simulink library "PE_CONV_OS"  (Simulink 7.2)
settings: Solver=ode45  SolverMode=SingleTasking  StartTime=0.0  StopTime=10.0  RelTol=1e-3
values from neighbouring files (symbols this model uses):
  C = 10e-3*1    (= 0.01)    [INIT_B6_2L_3Ph_IGBT_OS.m]    (also in INIT_B6_3L_3Ph_IGBT_OS.m; INIT_MMC_100L.m = 0.005; INIT_MMC_200L.m = 0.005; INIT_MMC_20L.m)
  FS = 900    [INIT_B6_2L_3Ph_IGBT_OS.m]    (also in INIT_B6_3L_3Ph_IGBT_OS.m; INIT_PWM_2L.m = 1000; INIT_PWM_3L.m = 1000; INIT_PWM_Con.m = 1000)
  LN = 2e-3    (= 0.002)    [INIT_PWM_2L.m]    (also in INIT_PWM_3L.m; INIT_PWM_Con.m; INIT_MMC_100L.m = 0.025; INIT_MMC_200L.m = 0.025)
  LS = 1e-3    (= 0.001)    [INIT_B6_2L_3Ph_IGBT_OS.m]    (also in INIT_B6_3L_3Ph_IGBT_OS.m; INIT_MMC_100L.m = 0.025; INIT_MMC_200L.m = 0.025; INIT_MMC_20L.m = 0.0025)
  LT = LN    (= 0.025)    [INIT_MMC_100L.m]    (also in INIT_MMC_200L.m; INIT_MMC_20L.m = 0.002; INIT_MMC_400L.m)
  Nc = 100    [INIT_MMC_100L.m]    (also in INIT_MMC_200L.m = 200; INIT_MMC_20L.m = 20; INIT_MMC_400L.m = 400)
  NT = sqrt(3)*340/400    [INIT_MMC_100L.m]    (also in INIT_MMC_200L.m; INIT_MMC_20L.m = sqrt(3); INIT_MMC_400L.m)
  Rg = 1e-3    (= 0.001)    [INIT_MMC_100L.m]    (also in INIT_MMC_200L.m; INIT_MMC_20L.m; INIT_MMC_400L.m)
  RN = 0.1    [INIT_PWM_2L.m]    (also in INIT_PWM_3L.m; INIT_PWM_Con.m; INIT_MMC_100L.m; INIT_MMC_200L.m)
  RT = RN    (= 0.1)    [INIT_MMC_100L.m]    (also in INIT_MMC_200L.m; INIT_MMC_20L.m; INIT_MMC_400L.m)
  UC0 = 600    [INIT_B6_2L_3Ph_IGBT_OS.m]    (also in INIT_B6_3L_3Ph_IGBT_OS.m = 500; INIT_MMC_100L.m = 6800; INIT_MMC_200L.m = 3400; INIT_MMC_20L.m = 5000)
undefined symbols (not defined in the file or in its folder): A, DT, FT, L, O1, O2, PHT, T, Td
libraries: simulink_extras x2
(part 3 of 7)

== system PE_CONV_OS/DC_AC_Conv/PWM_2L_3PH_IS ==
  Sw : Inport  OutDataType=sfix(16)  OutScaling=2^0
  vDC : Inport  Port=2  OutDataType=sfix(16)  OutScaling=2^0
  I_AB : Inport  Port=3  OutDataType=sfix(16)  OutScaling=2^0
  Mux : Mux  Inputs="[6  1  2]"
  pwm2l_IS_OS : S-Function  FunctionName=s_pwm_2L_3PH_IS_OS  Parameters=0  EnableBusSupport=off
  vABC : Outport  OutDataType=sfix(16)  OutScaling=2^0
  iABC : Outport  Port=2  OutDataType=sfix(16)  OutScaling=2^0
  vAB : Outport  Port=3  OutDataType=sfix(16)  OutScaling=2^0
  iT1,iD1,vT1 : Outport  Port=4  OutDataType=sfix(16)  OutScaling=2^0
  iDC : Outport  Port=5  OutDataType=sfix(16)  OutScaling=2^0
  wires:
  pwm2l_IS_OS/5 -> iDC/1
  pwm2l_IS_OS/3 -> vAB/1
  pwm2l_IS_OS/2 -> iABC/1
  pwm2l_IS_OS/1 -> vABC/1
  pwm2l_IS_OS/4 -> iT1,iD1,vT1/1
  I_AB/1 -> Mux/3
  Mux/1 -> pwm2l_IS_OS/1
  vDC/1 -> Mux/2
  Sw/1 -> Mux/1

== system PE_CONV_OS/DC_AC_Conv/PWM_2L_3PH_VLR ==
  Sw : Inport  OutDataType=sfix(16)  OutScaling=2^0
  vDC : Inport  Port=2  OutDataType=sfix(16)  OutScaling=2^0
  E_ABC : Inport  Port=3  OutDataType=sfix(16)  OutScaling=2^0
  Mux : Mux  Inputs="[6  1  3]"
  pwm2l_VLR_OS : S-Function  FunctionName=s_pwm_2L_3PH_VLR_OS  Parameters="[RL  LL]"  EnableBusSupport=off
  vABC : Outport  OutDataType=sfix(16)  OutScaling=2^0
  iABC : Outport  Port=2  OutDataType=sfix(16)  OutScaling=2^0
  vAB : Outport  Port=3  OutDataType=sfix(16)  OutScaling=2^0
  iT1,iD1,vT1 : Outport  Port=4  OutDataType=sfix(16)  OutScaling=2^0
  iDC : Outport  Port=5  OutDataType=sfix(16)  OutScaling=2^0
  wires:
  Sw/1 -> Mux/1
  vDC/1 -> Mux/2
  Mux/1 -> pwm2l_VLR_OS/1
  E_ABC/1 -> Mux/3
  pwm2l_VLR_OS/4 -> iT1,iD1,vT1/1
  pwm2l_VLR_OS/1 -> vABC/1
  pwm2l_VLR_OS/2 -> iABC/1
  pwm2l_VLR_OS/3 -> vAB/1
  pwm2l_VLR_OS/5 -> iDC/1

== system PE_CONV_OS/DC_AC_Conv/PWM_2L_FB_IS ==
  Sw : Inport  OutDataType=sfix(16)  OutScaling=2^0
  vDC : Inport  Port=2  OutDataType=sfix(16)  OutScaling=2^0
  IS : Inport  Port=3  OutDataType=sfix(16)  OutScaling=2^0
  Mux : Mux  Inputs="[4  1  1]"
  pwm2l_FB_IS_OS : S-Function  FunctionName=s_pwm_2L_FB_IS_OS  Parameters=0  EnableBusSupport=off
  vA : Outport  OutDataType=sfix(16)  OutScaling=2^0
  iA : Outport  Port=2  OutDataType=sfix(16)  OutScaling=2^0
  vAB : Outport  Port=3  OutDataType=sfix(16)  OutScaling=2^0
  iT1,iD1,vT1 : Outport  Port=4  OutDataType=sfix(16)  OutScaling=2^0
  iDC : Outport  Port=5  OutDataType=sfix(16)  OutScaling=2^0
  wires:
  pwm2l_FB_IS_OS/5 -> iDC/1
  Sw/1 -> Mux/1
  vDC/1 -> Mux/2
  Mux/1 -> pwm2l_FB_IS_OS/1
  IS/1 -> Mux/3
  pwm2l_FB_IS_OS/1 -> vA/1
  pwm2l_FB_IS_OS/2 -> iA/1
  pwm2l_FB_IS_OS/3 -> vAB/1
  pwm2l_FB_IS_OS/4 -> iT1,iD1,vT1/1

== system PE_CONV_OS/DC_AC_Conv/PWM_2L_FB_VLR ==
  Sw : Inport  OutDataType=sfix(16)  OutScaling=2^0
  vDC : Inport  Port=2  OutDataType=sfix(16)  OutScaling=2^0
  EA : Inport  Port=3  OutDataType=sfix(16)  OutScaling=2^0
  Mux : Mux  Inputs="[4  1  1]"
  pwm2l_FB_IS_OS : S-Function  FunctionName=s_pwm_2L_FB_VLR_OS  Parameters="[RL  LL]"  EnableBusSupport=off
  vA : Outport  OutDataType=sfix(16)  OutScaling=2^0
  iA1 : Outport  Port=2  OutDataType=sfix(16)  OutScaling=2^0
  vAB : Outport  Port=3  OutDataType=sfix(16)  OutScaling=2^0
  iT1,iD1,vT1 : Outport  Port=4  OutDataType=sfix(16)  OutScaling=2^0
  iDC : Outport  Port=5  OutDataType=sfix(16)  OutScaling=2^0
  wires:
  pwm2l_FB_IS_OS/5 -> iDC/1
  Sw/1 -> Mux/1
  vDC/1 -> Mux/2
  Mux/1 -> pwm2l_FB_IS_OS/1
  EA/1 -> Mux/3
  pwm2l_FB_IS_OS/1 -> vA/1
  pwm2l_FB_IS_OS/2 -> iA1/1
  pwm2l_FB_IS_OS/3 -> vAB/1
  pwm2l_FB_IS_OS/4 -> iT1,iD1,vT1/1

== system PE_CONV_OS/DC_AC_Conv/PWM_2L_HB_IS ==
  Sw : Inport  OutDataType=sfix(16)  OutScaling=2^0
  vDC : Inport  Port=2  OutDataType=sfix(16)  OutScaling=2^0
  IS : Inport  Port=3  OutDataType=sfix(16)  OutScaling=2^0
  Mux : Mux  Inputs="[2  1  1]"
  pwm2l_HB_IS_OS : S-Function  FunctionName=s_pwm_2L_HB_IS_OS  Parameters=0  EnableBusSupport=off
  vA : Outport  OutDataType=sfix(16)  OutScaling=2^0
  iA : Outport  Port=2  OutDataType=sfix(16)  OutScaling=2^0
  iT1,iD1,vT1 : Outport  Port=3  OutDataType=sfix(16)  OutScaling=2^0
  iDC : Outport  Port=4  OutDataType=sfix(16)  OutScaling=2^0
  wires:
  Sw/1 -> Mux/1
  vDC/1 -> Mux/2
  Mux/1 -> pwm2l_HB_IS_OS/1
  IS/1 -> Mux/3
  pwm2l_HB_IS_OS/1 -> vA/1
  pwm2l_HB_IS_OS/2 -> iA/1
  pwm2l_HB_IS_OS/3 -> iT1,iD1,vT1/1
  pwm2l_HB_IS_OS/4 -> iDC/1

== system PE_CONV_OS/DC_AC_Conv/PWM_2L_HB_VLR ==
  Sw : Inport  OutDataType=sfix(16)  OutScaling=2^0
  vDC : Inport  Port=2  OutDataType=sfix(16)  OutScaling=2^0
  EA : Inport  Port=3  OutDataType=sfix(16)  OutScaling=2^0
  Mux : Mux  Inputs="[2  1  1]"
  pwm2l_HB_VLR_OS : S-Function  FunctionName=s_pwm_2L_HB_VLR_OS  Parameters="[RL  LL]"  EnableBusSupport=off
  vA : Outport  OutDataType=sfix(16)  OutScaling=2^0
  iA : Outport  Port=2  OutDataType=sfix(16)  OutScaling=2^0
  iT1,iD1,vT1 : Outport  Port=3  OutDataType=sfix(16)  OutScaling=2^0
  iDC : Outport  Port=4  OutDataType=sfix(16)  OutScaling=2^0
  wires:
  Sw/1 -> Mux/1
  vDC/1 -> Mux/2
  Mux/1 -> pwm2l_HB_VLR_OS/1
  EA/1 -> Mux/3
  pwm2l_HB_VLR_OS/1 -> vA/1
  pwm2l_HB_VLR_OS/2 -> iA/1
  pwm2l_HB_VLR_OS/3 -> iT1,iD1,vT1/1
  pwm2l_HB_VLR_OS/4 -> iDC/1

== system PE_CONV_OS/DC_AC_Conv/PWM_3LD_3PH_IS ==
  Sw : Inport  OutDataType=sfix(16)  OutScaling=2^0
  vDC : Inport  Port=2  OutDataType=sfix(16)  OutScaling=2^0
  I_AB : Inport  Port=3  OutDataType=sfix(16)  OutScaling=2^0
  Mux : Mux  Inputs="[12  1  2]"
  pwm3LD_OS : S-Function  FunctionName=s_pwm_3LD_3PH_IS_OS  Parameters=0  EnableBusSupport=off
  vABC : Outport  OutDataType=sfix(16)  OutScaling=2^0
  iABC : Outport  Port=2  OutDataType=sfix(16)  OutScaling=2^0
  vAB : Outport  Port=3  OutDataType=sfix(16)  OutScaling=2^0
  "iT1, iD1,vT1" : Outport  Port=4  OutDataType=sfix(16)  OutScaling=2^0
  "iT2, iD2,vT2" : Outport  Port=5  OutDataType=sfix(16)  OutScaling=2^0
  iD5,vD5 : Outport  Port=6  OutDataType=sfix(16)  OutScaling=2^0
  iDC1,iDC2 : Outport  Port=7  OutDataType=sfix(16)  OutScaling=2^0
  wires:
  pwm3LD_OS/7 -> iDC1,iDC2/1
  pwm3LD_OS/6 -> iD5,vD5/1
  pwm3LD_OS/5 -> "iT2, iD2,vT2"/1
  pwm3LD_OS/3 -> vAB/1
  pwm3LD_OS/2 -> iABC/1
  pwm3LD_OS/4 -> "iT1, iD1,vT1"/1
  pwm3LD_OS/1 -> vABC/1
  I_AB/1 -> Mux/3
  Mux/1 -> pwm3LD_OS/1
  vDC/1 -> Mux/2
  Sw/1 -> Mux/1

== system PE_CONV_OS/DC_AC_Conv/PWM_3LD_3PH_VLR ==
  Sw : Inport  OutDataType=sfix(16)  OutScaling=2^0
  vDC : Inport  Port=2  OutDataType=sfix(16)  OutScaling=2^0
  E_ABC : Inport  Port=3  OutDataType=sfix(16)  OutScaling=2^0
  Mux : Mux  Inputs="[12 1  3]"
  pwm3LD_3PH_VLR_OS : S-Function  FunctionName=s_pwm_3LD_3PH_VLR_OS  Parameters="[RL  LL]"  EnableBusSupport=off
  vABC : Outport  OutDataType=sfix(16)  OutScaling=2^0
  iABC : Outport  Port=2  OutDataType=sfix(16)  OutScaling=2^0
  vAB : Outport  Port=3  OutDataType=sfix(16)  OutScaling=2^0
  "iT1, iD1,vT1" : Outport  Port=4  OutDataType=sfix(16)  OutScaling=2^0
  "iT2, iD2,vT2" : Outport  Port=5  OutDataType=sfix(16)  OutScaling=2^0
  iD5,vD5 : Outport  Port=6  OutDataType=sfix(16)  OutScaling=2^0
  iDC1,iDC2 : Outport  Port=7  OutDataType=sfix(16)  OutScaling=2^0
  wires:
  Sw/1 -> Mux/1
  vDC/1 -> Mux/2
  Mux/1 -> pwm3LD_3PH_VLR_OS/1
  E_ABC/1 -> Mux/3
  pwm3LD_3PH_VLR_OS/1 -> vABC/1
  pwm3LD_3PH_VLR_OS/4 -> "iT1, iD1,vT1"/1
  pwm3LD_3PH_VLR_OS/2 -> iABC/1
  pwm3LD_3PH_VLR_OS/3 -> vAB/1
  pwm3LD_3PH_VLR_OS/5 -> "iT2, iD2,vT2"/1
  pwm3LD_3PH_VLR_OS/6 -> iD5,vD5/1
  pwm3LD_3PH_VLR_OS/7 -> iDC1,iDC2/1

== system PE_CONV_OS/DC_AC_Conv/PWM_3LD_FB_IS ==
  Sw : Inport  OutDataType=sfix(16)  OutScaling=2^0
  vDC : Inport  Port=2  OutDataType=sfix(16)  OutScaling=2^0
  iS : Inport  Port=3  OutDataType=sfix(16)  OutScaling=2^0
  Mux : Mux  Inputs="[8  1  1]"
  pwm3LD_IS_OS : S-Function  FunctionName=s_pwm_3LD_FB_IS_OS  Parameters=0  EnableBusSupport=off
  vA : Outport  OutDataType=sfix(16)  OutScaling=2^0
  iA : Outport  Port=2  OutDataType=sfix(16)  OutScaling=2^0
  vAB : Outport  Port=3  OutDataType=sfix(16)  OutScaling=2^0
  "iT1, iD1,vT1" : Outport  Port=4  OutDataType=sfix(16)  OutScaling=2^0
  "iT2, iD2,vT2" : Outport  Port=5  OutDataType=sfix(16)  OutScaling=2^0
  iD5,vD5 : Outport  Port=6  OutDataType=sfix(16)  OutScaling=2^0
  iDC1,iDC2 : Outport  Port=7  OutDataType=sfix(16)  OutScaling=2^0
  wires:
  pwm3LD_IS_OS/2 -> iA/1
  pwm3LD_IS_OS/3 -> vAB/1
  pwm3LD_IS_OS/4 -> "iT1, iD1,vT1"/1
  pwm3LD_IS_OS/5 -> "iT2, iD2,vT2"/1
  pwm3LD_IS_OS/6 -> iD5,vD5/1
  pwm3LD_IS_OS/7 -> iDC1,iDC2/1
  Sw/1 -> Mux/1
  vDC/1 -> Mux/2
  Mux/1 -> pwm3LD_IS_OS/1
  iS/1 -> Mux/3
  pwm3LD_IS_OS/1 -> vA/1

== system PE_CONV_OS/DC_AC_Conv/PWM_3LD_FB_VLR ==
  Sw : Inport  OutDataType=sfix(16)  OutScaling=2^0
  vDC : Inport  Port=2  OutDataType=sfix(16)  OutScaling=2^0
  E_A : Inport  Port=3  OutDataType=sfix(16)  OutScaling=2^0
  Mux : Mux  Inputs="[8  1  1]"
  pwm3LD_VLR_OS : S-Function  FunctionName=s_pwm_3LD_FB_VLR_OS  Parameters="[RL  LL]"  EnableBusSupport=off
  vA : Outport  OutDataType=sfix(16)  OutScaling=2^0
  iA : Outport  Port=2  OutDataType=sfix(16)  OutScaling=2^0
  vAB : Outport  Port=3  OutDataType=sfix(16)  OutScaling=2^0
  "iT1, iD1,vT1" : Outport  Port=4  OutDataType=sfix(16)  OutScaling=2^0
  "iT2, iD2,vT2" : Outport  Port=5  OutDataType=sfix(16)  OutScaling=2^0
  iD5,vD5 : Outport  Port=6  OutDataType=sfix(16)  OutScaling=2^0
  iDC1,iDC2 : Outport  Port=7  OutDataType=sfix(16)  OutScaling=2^0
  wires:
  pwm3LD_VLR_OS/7 -> iDC1,iDC2/1
  pwm3LD_VLR_OS/6 -> iD5,vD5/1
  pwm3LD_VLR_OS/5 -> "iT2, iD2,vT2"/1
  pwm3LD_VLR_OS/4 -> "iT1, iD1,vT1"/1
  pwm3LD_VLR_OS/3 -> vAB/1
  pwm3LD_VLR_OS/2 -> iA/1
  pwm3LD_VLR_OS/1 -> vA/1
  E_A/1 -> Mux/3
  Mux/1 -> pwm3LD_VLR_OS/1
  vDC/1 -> Mux/2
  Sw/1 -> Mux/1

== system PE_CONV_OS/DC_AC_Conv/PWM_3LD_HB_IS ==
  Sw : Inport  OutDataType=sfix(16)  OutScaling=2^0
  vDC : Inport  Port=2  OutDataType=sfix(16)  OutScaling=2^0
  iS : Inport  Port=3  OutDataType=sfix(16)  OutScaling=2^0
  Mux : Mux  Inputs="[4  1  1]"
  pwm3LD_HB_IS_OS : S-Function  FunctionName=s_pwm_3LD_HB_IS_OS  Parameters=0  EnableBusSupport=off
  vA : Outport  OutDataType=sfix(16)  OutScaling=2^0
  iA : Outport  Port=2  OutDataType=sfix(16)  OutScaling=2^0
  "iT1, iD1,vT1" : Outport  Port=3  OutDataType=sfix(16)  OutScaling=2^0
  "iT2, iD2,vT2" : Outport  Port=4  OutDataType=sfix(16)  OutScaling=2^0
  iD5,vD5 : Outport  Port=5  OutDataType=sfix(16)  OutScaling=2^0
  iDC1,iDC2 : Outport  Port=6  OutDataType=sfix(16)  OutScaling=2^0
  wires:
  pwm3LD_HB_IS_OS/6 -> iDC1,iDC2/1
  pwm3LD_HB_IS_OS/1 -> vA/1
  iS/1 -> Mux/3
  Mux/1 -> pwm3LD_HB_IS_OS/1
  vDC/1 -> Mux/2
  Sw/1 -> Mux/1
  pwm3LD_HB_IS_OS/2 -> iA/1
  pwm3LD_HB_IS_OS/3 -> "iT1, iD1,vT1"/1
  pwm3LD_HB_IS_OS/4 -> "iT2, iD2,vT2"/1
  pwm3LD_HB_IS_OS/5 -> iD5,vD5/1

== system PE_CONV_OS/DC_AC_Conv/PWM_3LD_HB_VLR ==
  Sw : Inport  OutDataType=sfix(16)  OutScaling=2^0
  vDC : Inport  Port=2  OutDataType=sfix(16)  OutScaling=2^0
  EA : Inport  Port=3  OutDataType=sfix(16)  OutScaling=2^0
  Mux : Mux  Inputs="[4  1 1]"
  pwm3LD_HB_VLR_OS : S-Function  FunctionName=s_pwm_3LD_HB_VLR_OS  Parameters="[RL  LL]"  EnableBusSupport=off
  vA : Outport  OutDataType=sfix(16)  OutScaling=2^0
  iA : Outport  Port=2  OutDataType=sfix(16)  OutScaling=2^0
  "iT1, iD1,vT1" : Outport  Port=3  OutDataType=sfix(16)  OutScaling=2^0
  "iT2, iD2,vT2" : Outport  Port=4  OutDataType=sfix(16)  OutScaling=2^0
  iD5,vD5 : Outport  Port=5  OutDataType=sfix(16)  OutScaling=2^0
  iDC1,iDC2 : Outport  Port=6  OutDataType=sfix(16)  OutScaling=2^0
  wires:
  Sw/1 -> Mux/1
  vDC/1 -> Mux/2
  Mux/1 -> pwm3LD_HB_VLR_OS/1
  EA/1 -> Mux/3
  pwm3LD_HB_VLR_OS/1 -> vA/1
  pwm3LD_HB_VLR_OS/2 -> iA/1
  pwm3LD_HB_VLR_OS/3 -> "iT1, iD1,vT1"/1
  pwm3LD_HB_VLR_OS/4 -> "iT2, iD2,vT2"/1
  pwm3LD_HB_VLR_OS/5 -> iD5,vD5/1
  pwm3LD_HB_VLR_OS/6 -> iDC1,iDC2/1

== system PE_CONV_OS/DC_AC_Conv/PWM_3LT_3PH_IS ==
  Sw : Inport  OutDataType=sfix(16)  OutScaling=2^0
  vDC : Inport  Port=2  OutDataType=sfix(16)  OutScaling=2^0
  I_AB : Inport  Port=3  OutDataType=sfix(16)  OutScaling=2^0
  Mux : Mux  Inputs="[12  1  2]"
  pwm3LD_OS : S-Function  FunctionName=s_pwm_3LT_3PH_IS_OS  Parameters=0  EnableBusSupport=off
  vABC : Outport  OutDataType=sfix(16)  OutScaling=2^0
  iABC : Outport  Port=2  OutDataType=sfix(16)  OutScaling=2^0
  vAB : Outport  Port=3  OutDataType=sfix(16)  OutScaling=2^0
  "iT1, iD1,vT1" : Outport  Port=4  OutDataType=sfix(16)  OutScaling=2^0
  "iT2, iD2,vT2" : Outport  Port=5  OutDataType=sfix(16)  OutScaling=2^0
  iDC1,iDC2 : Outport  Port=6  OutDataType=sfix(16)  OutScaling=2^0
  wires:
  Sw/1 -> Mux/1
  vDC/1 -> Mux/2
  Mux/1 -> pwm3LD_OS/1
  I_AB/1 -> Mux/3
  pwm3LD_OS/1 -> vABC/1
  pwm3LD_OS/4 -> "iT1, iD1,vT1"/1
  pwm3LD_OS/2 -> iABC/1
  pwm3LD_OS/3 -> vAB/1
  pwm3LD_OS/5 -> "iT2, iD2,vT2"/1
  pwm3LD_OS/6 -> iDC1,iDC2/1

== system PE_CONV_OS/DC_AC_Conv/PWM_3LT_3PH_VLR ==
  Sw : Inport  OutDataType=sfix(16)  OutScaling=2^0
  vDC : Inport  Port=2  OutDataType=sfix(16)  OutScaling=2^0
  E_ABC : Inport  Port=3  OutDataType=sfix(16)  OutScaling=2^0
  Mux : Mux  Inputs="[12 1  3]"
  pwm3LD_3PH_VLR_OS : S-Function  FunctionName=s_pwm_3LT_3PH_VLR_OS  Parameters="[RL  LL]"  EnableBusSupport=off
  vABC : Outport  OutDataType=sfix(16)  OutScaling=2^0
  iABC : Outport  Port=2  OutDataType=sfix(16)  OutScaling=2^0
  vAB : Outport  Port=3  OutDataType=sfix(16)  OutScaling=2^0
  "iT1, iD1,vT1" : Outport  Port=4  OutDataType=sfix(16)  OutScaling=2^0
  "iT2, iD2,vT2" : Outport  Port=5  OutDataType=sfix(16)  OutScaling=2^0
  iDC1,iDC2 : Outport  Port=6  OutDataType=sfix(16)  OutScaling=2^0
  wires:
  pwm3LD_3PH_VLR_OS/6 -> iDC1,iDC2/1
  pwm3LD_3PH_VLR_OS/5 -> "iT2, iD2,vT2"/1
  pwm3LD_3PH_VLR_OS/3 -> vAB/1
  pwm3LD_3PH_VLR_OS/2 -> iABC/1
  pwm3LD_3PH_VLR_OS/4 -> "iT1, iD1,vT1"/1
  pwm3LD_3PH_VLR_OS/1 -> vABC/1
  E_ABC/1 -> Mux/3
  Mux/1 -> pwm3LD_3PH_VLR_OS/1
  vDC/1 -> Mux/2
  Sw/1 -> Mux/1

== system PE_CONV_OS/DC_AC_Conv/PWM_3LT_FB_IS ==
  Sw : Inport  OutDataType=sfix(16)  OutScaling=2^0
  vDC : Inport  Port=2  OutDataType=sfix(16)  OutScaling=2^0
  IS : Inport  Port=3  OutDataType=sfix(16)  OutScaling=2^0
  Mux : Mux  Inputs="[8 1  1]"
  pwm3LD_IS_OS : S-Function  FunctionName=s_pwm_3LT_FB_IS_OS  Parameters=[0]  EnableBusSupport=off
  vA : Outport  OutDataType=sfix(16)  OutScaling=2^0
  IA : Outport  Port=2  OutDataType=sfix(16)  OutScaling=2^0
  vAB : Outport  Port=3  OutDataType=sfix(16)  OutScaling=2^0
  "iT1, iD1,vT1" : Outport  Port=4  OutDataType=sfix(16)  OutScaling=2^0
  "iT2, iD2,vT2" : Outport  Port=5  OutDataType=sfix(16)  OutScaling=2^0
  iDC1,iDC2 : Outport  Port=6  OutDataType=sfix(16)  OutScaling=2^0
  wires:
  pwm3LD_IS_OS/6 -> iDC1,iDC2/1
  pwm3LD_IS_OS/5 -> "iT2, iD2,vT2"/1
  pwm3LD_IS_OS/4 -> "iT1, iD1,vT1"/1
  pwm3LD_IS_OS/3 -> vAB/1
  pwm3LD_IS_OS/2 -> IA/1
  Sw/1 -> Mux/1
  vDC/1 -> Mux/2
  Mux/1 -> pwm3LD_IS_OS/1
  IS/1 -> Mux/3
  pwm3LD_IS_OS/1 -> vA/1

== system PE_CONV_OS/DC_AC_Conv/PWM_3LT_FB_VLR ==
  Sw : Inport  OutDataType=sfix(16)  OutScaling=2^0
  vDC : Inport  Port=2  OutDataType=sfix(16)  OutScaling=2^0
  E_A : Inport  Port=3  OutDataType=sfix(16)  OutScaling=2^0
  Mux : Mux  Inputs="[8  1  1]"
  pwm3LD_VLR_OS : S-Function  FunctionName=s_pwm_3LT_FB_VLR_OS  Parameters="[RL  LL]"  EnableBusSupport=off
  vA : Outport  OutDataType=sfix(16)  OutScaling=2^0
  iA : Outport  Port=2  OutDataType=sfix(16)  OutScaling=2^0
  vAB : Outport  Port=3  OutDataType=sfix(16)  OutScaling=2^0
  "iT1, iD1,vT1" : Outport  Port=4  OutDataType=sfix(16)  OutScaling=2^0
  "iT2, iD2,vT2" : Outport  Port=5  OutDataType=sfix(16)  OutScaling=2^0
  "iDC1, iDC2" : Outport  Port=6  OutDataType=sfix(16)  OutScaling=2^0
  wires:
  pwm3LD_VLR_OS/6 -> "iDC1, iDC2"/1
  Sw/1 -> Mux/1
  vDC/1 -> Mux/2
  Mux/1 -> pwm3LD_VLR_OS/1
  E_A/1 -> Mux/3
  pwm3LD_VLR_OS/1 -> vA/1
  pwm3LD_VLR_OS/2 -> iA/1
  pwm3LD_VLR_OS/3 -> vAB/1
  pwm3LD_VLR_OS/4 -> "iT1, iD1,vT1"/1
  pwm3LD_VLR_OS/5 -> "iT2, iD2,vT2"/1

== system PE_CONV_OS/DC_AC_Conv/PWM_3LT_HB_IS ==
  Sw : Inport  OutDataType=sfix(16)  OutScaling=2^0
  vDC : Inport  Port=2  OutDataType=sfix(16)  OutScaling=2^0
  iS : Inport  Port=3  OutDataType=sfix(16)  OutScaling=2^0
  Mux : Mux  Inputs="[4  1  1]"
  pwm3LT_HB_IS_OS : S-Function  FunctionName=s_pwm_3LT_HB_IS_OS  Parameters=0  EnableBusSupport=off
  vA : Outport  OutDataType=sfix(16)  OutScaling=2^0
  iA : Outport  Port=2  OutDataType=sfix(16)  OutScaling=2^0
  "iT1, iD1,vT1" : Outport  Port=3  OutDataType=sfix(16)  OutScaling=2^0
  "iT2, iD2,vT2" : Outport  Port=4  OutDataType=sfix(16)  OutScaling=2^0
  iDC1,iDC2 : Outport  Port=5  OutDataType=sfix(16)  OutScaling=2^0
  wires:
  pwm3LT_HB_IS_OS/5 -> iDC1,iDC2/1
  pwm3LT_HB_IS_OS/4 -> "iT2, iD2,vT2"/1
  pwm3LT_HB_IS_OS/3 -> "iT1, iD1,vT1"/1
  pwm3LT_HB_IS_OS/2 -> iA/1
  Sw/1 -> Mux/1
  vDC/1 -> Mux/2
  Mux/1 -> pwm3LT_HB_IS_OS/1
  iS/1 -> Mux/3
  pwm3LT_HB_IS_OS/1 -> vA/1

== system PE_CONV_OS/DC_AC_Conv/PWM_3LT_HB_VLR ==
  Sw : Inport  OutDataType=sfix(16)  OutScaling=2^0
  vDC : Inport  Port=2  OutDataType=sfix(16)  OutScaling=2^0
  EA : Inport  Port=3  OutDataType=sfix(16)  OutScaling=2^0
  Mux : Mux  Inputs="[4  1 1]"
  pwm3LD_HB_VLR_OS : S-Function  FunctionName=s_pwm_3LT_HB_VLR_OS  Parameters="[RL  LL]"  EnableBusSupport=off
  vA : Outport  OutDataType=sfix(16)  OutScaling=2^0
  iA : Outport  Port=2  OutDataType=sfix(16)  OutScaling=2^0
  "iT1, iD1,vT1" : Outport  Port=3  OutDataType=sfix(16)  OutScaling=2^0
  "iT2, iD2,vT2" : Outport  Port=4  OutDataType=sfix(16)  OutScaling=2^0
  iDC1,iDC2 : Outport  Port=5  OutDataType=sfix(16)  OutScaling=2^0
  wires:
  pwm3LD_HB_VLR_OS/5 -> iDC1,iDC2/1
  pwm3LD_HB_VLR_OS/4 -> "iT2, iD2,vT2"/1
  pwm3LD_HB_VLR_OS/3 -> "iT1, iD1,vT1"/1
  pwm3LD_HB_VLR_OS/2 -> iA/1
  pwm3LD_HB_VLR_OS/1 -> vA/1
  EA/1 -> Mux/3
  Mux/1 -> pwm3LD_HB_VLR_OS/1
  vDC/1 -> Mux/2
  Sw/1 -> Mux/1

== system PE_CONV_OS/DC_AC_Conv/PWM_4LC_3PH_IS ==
  Sw : Inport  OutDataType=sfix(16)  OutScaling=2^0
  vDC : Inport  Port=2  OutDataType=sfix(16)  OutScaling=2^0
  i_AB : Inport  Port=3  OutDataType=sfix(16)  OutScaling=2^0
  Mux : Mux  Inputs="[18  1  2]"
  pwm3LD_3PH_IS_OS : S-Function  FunctionName=s_pwm_4LC_3PH_IS_OS  Parameters="[C1  VC10  C2  VC20]"  EnableBusSupport=off
  vABC : Outport  OutDataType=sfix(16)  OutScaling=2^0
  iABC : Outport  Port=2  OutDataType=sfix(16)  OutScaling=2^0
  vAB : Outport  Port=3  OutDataType=sfix(16)  OutScaling=2^0
  iT1,iD1,vT1 : Outport  Port=4  OutDataType=sfix(16)  OutScaling=2^0
  iT2,ID2,vT2 : Outport  Port=5  OutDataType=sfix(16)  OutScaling=2^0
  iT3,iD3,vT3 : Outport  Port=6  OutDataType=sfix(16)  OutScaling=2^0
  iDC1,IDC2 : Outport  Port=7  OutDataType=sfix(16)  OutScaling=2^0
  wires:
  pwm3LD_3PH_IS_OS/6 -> iT3,iD3,vT3/1
  pwm3LD_3PH_IS_OS/5 -> iT2,ID2,vT2/1
  pwm3LD_3PH_IS_OS/4 -> iT1,iD1,vT1/1
  pwm3LD_3PH_IS_OS/3 -> vAB/1
  Sw/1 -> Mux/1
  vDC/1 -> Mux/2
  Mux/1 -> pwm3LD_3PH_IS_OS/1
  i_AB/1 -> Mux/3
  pwm3LD_3PH_IS_OS/1 -> vABC/1
  pwm3LD_3PH_IS_OS/2 -> iABC/1
  pwm3LD_3PH_IS_OS/7 -> iDC1,IDC2/1

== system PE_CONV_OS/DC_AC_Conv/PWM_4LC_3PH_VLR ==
  Sw : Inport  OutDataType=sfix(16)  OutScaling=2^0
  vDC : Inport  Port=2  OutDataType=sfix(16)  OutScaling=2^0
  E_ABC : Inport  Port=3  OutDataType=sfix(16)  OutScaling=2^0
  Mux : Mux  Inputs="[18  1  3]"
  pwm3LD_3PH_VLR_OS : S-Function  FunctionName=s_pwm_4LC_3PH_VLR_OS  Parameters="[C1  VC10  C2  VC20  RL  LL]"  EnableBusSupport=off
  vABC : Outport  OutDataType=sfix(16)  OutScaling=2^0
  iABC : Outport  Port=2  OutDataType=sfix(16)  OutScaling=2^0
  vAB : Outport  Port=3  OutDataType=sfix(16)  OutScaling=2^0
  iT1,iD1,vT1 : Outport  Port=4  OutDataType=sfix(16)  OutScaling=2^0
  iT2,ID2,vT2 : Outport  Port=5  OutDataType=sfix(16)  OutScaling=2^0
  iT3,iD3,vT3 : Outport  Port=6  OutDataType=sfix(16)  OutScaling=2^0
  iDC1. iDC2 : Outport  Port=7  OutDataType=sfix(16)  OutScaling=2^0
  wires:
  pwm3LD_3PH_VLR_OS/7 -> iDC1. iDC2/1
  pwm3LD_3PH_VLR_OS/2 -> iABC/1
  pwm3LD_3PH_VLR_OS/1 -> vABC/1
  E_ABC/1 -> Mux/3
  Mux/1 -> pwm3LD_3PH_VLR_OS/1
  vDC/1 -> Mux/2
  Sw/1 -> Mux/1
  pwm3LD_3PH_VLR_OS/3 -> vAB/1
  pwm3LD_3PH_VLR_OS/4 -> iT1,iD1,vT1/1
  pwm3LD_3PH_VLR_OS/5 -> iT2,ID2,vT2/1
  pwm3LD_3PH_VLR_OS/6 -> iT3,iD3,vT3/1

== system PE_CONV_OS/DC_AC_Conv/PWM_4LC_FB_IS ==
  Sw : Inport  OutDataType=sfix(16)  OutScaling=2^0
  vDC : Inport  Port=2  OutDataType=sfix(16)  OutScaling=2^0
  i_A : Inport  Port=3  OutDataType=sfix(16)  OutScaling=2^0
  Mux : Mux  Inputs="[12  1  1]"
  pwm4Lc_HB_IS_OS : S-Function  FunctionName=s_pwm_4LC_FB_IS_OS  Parameters="[C1  VC10  C2  VC20]"  EnableBusSupport=off
  vA : Outport  OutDataType=sfix(16)  OutScaling=2^0
  iA : Outport  Port=2  OutDataType=sfix(16)  OutScaling=2^0
  iT1,iD1,vT1 : Outport  Port=3  OutDataType=sfix(16)  OutScaling=2^0
  iT2,ID2,vT2 : Outport  Port=4  OutDataType=sfix(16)  OutScaling=2^0
  iT3,iD3,vT3 : Outport  Port=5  OutDataType=sfix(16)  OutScaling=2^0
  iDC1,IDC2 : Outport  Port=6  OutDataType=sfix(16)  OutScaling=2^0
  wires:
  pwm4Lc_HB_IS_OS/5 -> iT3,iD3,vT3/1
  pwm4Lc_HB_IS_OS/4 -> iT2,ID2,vT2/1
  pwm4Lc_HB_IS_OS/3 -> iT1,iD1,vT1/1
  Sw/1 -> Mux/1
  vDC/1 -> Mux/2
  Mux/1 -> pwm4Lc_HB_IS_OS/1
  i_A/1 -> Mux/3
  pwm4Lc_HB_IS_OS/1 -> vA/1
  pwm4Lc_HB_IS_OS/2 -> iA/1
  pwm4Lc_HB_IS_OS/6 -> iDC1,IDC2/1

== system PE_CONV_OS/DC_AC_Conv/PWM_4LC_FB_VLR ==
  Sw : Inport  OutDataType=sfix(16)  OutScaling=2^0
  vDC : Inport  Port=2  OutDataType=sfix(16)  OutScaling=2^0
  VL : Inport  Port=3  OutDataType=sfix(16)  OutScaling=2^0
  Mux : Mux  Inputs="[12  1  1]"
  pwm4Lc_HB_IS_OS : S-Function  FunctionName=s_pwm_4LC_FB_VLR_OS  Parameters="[C1  VC10  C2  VC20 R1 L1]"  EnableBusSupport=off
  vA : Outport  OutDataType=sfix(16)  OutScaling=2^0
  iA : Outport  Port=2  OutDataType=sfix(16)  OutScaling=2^0
  iT1,iD1,vT1 : Outport  Port=3  OutDataType=sfix(16)  OutScaling=2^0
  iT2,ID2,vT2 : Outport  Port=4  OutDataType=sfix(16)  OutScaling=2^0
  iT3,iD3,vT3 : Outport  Port=5  OutDataType=sfix(16)  OutScaling=2^0
  iDC1,IDC2 : Outport  Port=6  OutDataType=sfix(16)  OutScaling=2^0
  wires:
  pwm4Lc_HB_IS_OS/5 -> iT3,iD3,vT3/1
  pwm4Lc_HB_IS_OS/4 -> iT2,ID2,vT2/1
  pwm4Lc_HB_IS_OS/3 -> iT1,iD1,vT1/1
  Sw/1 -> Mux/1
  vDC/1 -> Mux/2
  Mux/1 -> pwm4Lc_HB_IS_OS/1
  VL/1 -> Mux/3
  pwm4Lc_HB_IS_OS/1 -> vA/1
  pwm4Lc_HB_IS_OS/2 -> iA/1
  pwm4Lc_HB_IS_OS/6 -> iDC1,IDC2/1

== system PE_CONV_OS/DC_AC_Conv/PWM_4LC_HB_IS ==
  Sw : Inport  OutDataType=sfix(16)  OutScaling=2^0
  vDC : Inport  Port=2  OutDataType=sfix(16)  OutScaling=2^0
  i_A : Inport  Port=3  OutDataType=sfix(16)  OutScaling=2^0
  Mux : Mux  Inputs="[6  1  1]"
  pwm4Lc_HB_IS_OS : S-Function  FunctionName=s_pwm_4LC_HB_IS_OS  Parameters="[C1  VC10  C2  VC20]"  EnableBusSupport=off
  vA : Outport  OutDataType=sfix(16)  OutScaling=2^0
  iA : Outport  Port=2  OutDataType=sfix(16)  OutScaling=2^0
  iT1,iD1,vT1 : Outport  Port=3  OutDataType=sfix(16)  OutScaling=2^0
  iT2,ID2,vT2 : Outport  Port=4  OutDataType=sfix(16)  OutScaling=2^0
  iT3,iD3,vT3 : Outport  Port=5  OutDataType=sfix(16)  OutScaling=2^0
  iDC1,IDC2 : Outport  Port=6  OutDataType=sfix(16)  OutScaling=2^0
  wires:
  pwm4Lc_HB_IS_OS/5 -> iT3,iD3,vT3/1
  pwm4Lc_HB_IS_OS/4 -> iT2,ID2,vT2/1
  pwm4Lc_HB_IS_OS/3 -> iT1,iD1,vT1/1
  Sw/1 -> Mux/1
  vDC/1 -> Mux/2
  Mux/1 -> pwm4Lc_HB_IS_OS/1
  i_A/1 -> Mux/3
  pwm4Lc_HB_IS_OS/1 -> vA/1
  pwm4Lc_HB_IS_OS/2 -> iA/1
  pwm4Lc_HB_IS_OS/6 -> iDC1,IDC2/1

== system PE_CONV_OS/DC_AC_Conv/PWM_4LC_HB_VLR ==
  Sw : Inport  OutDataType=sfix(16)  OutScaling=2^0
  vDC : Inport  Port=2  OutDataType=sfix(16)  OutScaling=2^0
  vL : Inport  Port=3  OutDataType=sfix(16)  OutScaling=2^0
  Mux : Mux  Inputs="[6  1  1]"
  pwm4Lc_HB_IS_OS : S-Function  FunctionName=s_pwm_4LC_HB_VLR_OS  Parameters="[C1  VC10  C2  VC20 R1  L1]"  EnableBusSupport=off
  vA : Outport  OutDataType=sfix(16)  OutScaling=2^0
  iA : Outport  Port=2  OutDataType=sfix(16)  OutScaling=2^0
  iT1,iD1,vT1 : Outport  Port=3  OutDataType=sfix(16)  OutScaling=2^0
  iT2,ID2,vT2 : Outport  Port=4  OutDataType=sfix(16)  OutScaling=2^0
  iT3,iD3,vT3 : Outport  Port=5  OutDataType=sfix(16)  OutScaling=2^0
  iDC1,IDC2 : Outport  Port=6  OutDataType=sfix(16)  OutScaling=2^0
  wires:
  pwm4Lc_HB_IS_OS/5 -> iT3,iD3,vT3/1
  pwm4Lc_HB_IS_OS/4 -> iT2,ID2,vT2/1
  pwm4Lc_HB_IS_OS/3 -> iT1,iD1,vT1/1
  Sw/1 -> Mux/1
  vDC/1 -> Mux/2
  Mux/1 -> pwm4Lc_HB_IS_OS/1
  vL/1 -> Mux/3
  pwm4Lc_HB_IS_OS/1 -> vA/1
  pwm4Lc_HB_IS_OS/2 -> iA/1
  pwm4Lc_HB_IS_OS/6 -> iDC1,IDC2/1

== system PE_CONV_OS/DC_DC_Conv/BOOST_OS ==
  sw : Inport  OutDataType=sfix(16)  OutScaling=2^0
  E : Inport  Port=2  OutDataType=sfix(16)  OutScaling=2^0
  IDC : Inport  Port=3  OutDataType=sfix(16)  OutScaling=2^0
  BOOST : S-Function  FunctionName=s_boost_OS  Parameters="[L1  IL0  C1   UC0  R1]"  EnableBusSupport=off
  Mux1 : Mux  Inputs=3
  iT1 : Outport  OutDataType=sfix(16)  OutScaling=2^0
  iD1 : Outport  Port=2  OutDataType=sfix(16)  OutScaling=2^0
  iL1 : Outport  Port=3  OutDataType=sfix(16)  OutScaling=2^0
  vC : Outport  Port=4  OutDataType=sfix(16)  OutScaling=2^0
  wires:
  IDC/1 -> Mux1/3
  BOOST/4 -> vC/1
  BOOST/3 -> iL1/1
  BOOST/2 -> iD1/1
  BOOST/1 -> iT1/1
  E/1 -> Mux1/2
  sw/1 -> Mux1/1
  Mux1/1 -> BOOST/1

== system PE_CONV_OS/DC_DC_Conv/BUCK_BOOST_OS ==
  sw : Inport  OutDataType=sfix(16)  OutScaling=2^0
  E : Inport  Port=2  OutDataType=sfix(16)  OutScaling=2^0
  IDC : Inport  Port=3  OutDataType=sfix(16)  OutScaling=2^0
  Mux1 : Mux  Inputs=3
  buck_boost : S-Function  FunctionName=s_Buck_boost_OS  Parameters="[L1  IL0  C1   UC0  R1]"  EnableBusSupport=off
  iT1 : Outport  OutDataType=sfix(16)  OutScaling=2^0
  iD1 : Outport  Port=2  OutDataType=sfix(16)  OutScaling=2^0
  iL1 : Outport  Port=3  OutDataType=sfix(16)  OutScaling=2^0
  vC : Outport  Port=4  OutDataType=sfix(16)  OutScaling=2^0
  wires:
  IDC/1 -> Mux1/3
  Mux1/1 -> buck_boost/1
  E/1 -> Mux1/2
  sw/1 -> Mux1/1
  buck_boost/4 -> vC/1
  buck_boost/3 -> iL1/1
  buck_boost/2 -> iD1/1
  buck_boost/1 -> iT1/1

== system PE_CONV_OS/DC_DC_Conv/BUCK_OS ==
  sw : Inport
  E : Inport  Port=2
  IDC : Inport  Port=3
  Mux1 : Mux  Inputs=3
  S_BUCK : S-Function  FunctionName=s_buck_OS  Parameters="[L1  IL0  C1   UC0  R1]"  EnableBusSupport=off
  iT1 : Outport
  iD1 : Outport  Port=2
  iL1 : Outport  Port=3
  vC : Outport  Port=4
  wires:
  Mux1/1 -> S_BUCK/1
  IDC/1 -> Mux1/3
  E/1 -> Mux1/2
  sw/1 -> Mux1/1
  S_BUCK/4 -> vC/1
  S_BUCK/3 -> iL1/1
  S_BUCK/2 -> iD1/1
  S_BUCK/1 -> iT1/1

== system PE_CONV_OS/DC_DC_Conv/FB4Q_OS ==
  sw : Inport  OutDataType=sfix(16)  OutScaling=2^0
  E : Inport  Port=2  OutDataType=sfix(16)  OutScaling=2^0
  ID : Inport  Port=3  OutDataType=sfix(16)  OutScaling=2^0
  FB4Q_DC_DC : S-Function  FunctionName=s_FB4Q_DC_OS  Parameters="[L  IL0  C  VC0   R]"  EnableBusSupport=off
  Mux1 : Mux  Inputs=3
  "iT1, iD1" : Outport  OutDataType=sfix(16)  OutScaling=2^0
  "iT3, iD3" : Outport  Port=2  OutDataType=sfix(16)  OutScaling=2^0
  vO : Outport  Port=3  OutDataType=sfix(16)  OutScaling=2^0
  iL : Outport  Port=4  OutDataType=sfix(16)  OutScaling=2^0
  vC : Outport  Port=5  OutDataType=sfix(16)  OutScaling=2^0
  iE : Outport  Port=6  OutDataType=sfix(16)  OutScaling=2^0
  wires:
  FB4Q_DC_DC/6 -> iE/1
  FB4Q_DC_DC/5 -> vC/1
  FB4Q_DC_DC/3 -> vO/1
  FB4Q_DC_DC/4 -> iL/1
  ID/1 -> Mux1/3
  FB4Q_DC_DC/2 -> "iT3, iD3"/1
  FB4Q_DC_DC/1 -> "iT1, iD1"/1
  E/1 -> Mux1/2
  sw/1 -> Mux1/1
  Mux1/1 -> FB4Q_DC_DC/1

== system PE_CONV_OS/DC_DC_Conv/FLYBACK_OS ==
  sw : Inport  OutDataType=sfix(16)  OutScaling=2^0
  E : Inport  Port=2  OutDataType=sfix(16)  OutScaling=2^0
  IDC : Inport  Port=3  OutDataType=sfix(16)  OutScaling=2^0
  Flyback : S-Function  FunctionName=s_flyback_OS  Parameters="[L1  L2   KP  C  UC0  R]"  EnableBusSupport=off
  Mux1 : Mux  Inputs=3
  iT1 : Outport  OutDataType=sfix(16)  OutScaling=2^0
  iD1 : Outport  Port=2  OutDataType=sfix(16)  OutScaling=2^0
  tL1 : Outport  Port=3  OutDataType=sfix(16)  OutScaling=2^0
  vL1,vL2 : Outport  Port=4  OutDataType=sfix(16)  OutScaling=2^0
  vC : Outport  Port=5  OutDataType=sfix(16)  OutScaling=2^0
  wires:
  IDC/1 -> Mux1/3
  Flyback/5 -> vC/1
  Flyback/4 -> vL1,vL2/1
  Flyback/3 -> tL1/1
  Flyback/2 -> iD1/1
  Flyback/1 -> iT1/1
  Mux1/1 -> Flyback/1
  E/1 -> Mux1/2
  sw/1 -> Mux1/1

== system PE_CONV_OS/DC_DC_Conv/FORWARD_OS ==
  sw : Inport  OutDataType=sfix(16)  OutScaling=2^0
  E : Inport  Port=2  OutDataType=sfix(16)  OutScaling=2^0
  IDC : Inport  Port=3  OutDataType=sfix(16)  OutScaling=2^0
  Forward1 : S-Function  FunctionName=s_forward_OS  Parameters="[L1  L2  L3   KP1  KP2  KP3  L C  UC0  R]"  EnableBusSupport=off
  Mux1 : Mux  Inputs=3
  iT1 : Outport  OutDataType=sfix(16)  OutScaling=2^0
  iD1 : Outport  Port=2  OutDataType=sfix(16)  OutScaling=2^0
  iL1 : Outport  Port=3  OutDataType=sfix(16)  OutScaling=2^0
  vL1,vL2,vL3 : Outport  Port=4  OutDataType=sfix(16)  OutScaling=2^0
  iD2 : Outport  Port=5  OutDataType=sfix(16)  OutScaling=2^0
  iD3 : Outport  Port=6  OutDataType=sfix(16)  OutScaling=2^0
  vC : Outport  Port=7  OutDataType=sfix(16)  OutScaling=2^0
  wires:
  Forward1/7 -> vC/1
  Forward1/5 -> iD2/1
  Forward1/4 -> vL1,vL2,vL3/1
  Forward1/3 -> iL1/1
  Forward1/2 -> iD1/1
  Forward1/1 -> iT1/1
  Forward1/6 -> iD3/1
  IDC/1 -> Mux1/3
  E/1 -> Mux1/2
  Mux1/1 -> Forward1/1
  sw/1 -> Mux1/1

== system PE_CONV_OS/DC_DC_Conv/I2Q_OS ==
  sw : Inport  OutDataType=sfix(16)  OutScaling=2^0
  E : Inport  Port=2  OutDataType=sfix(16)  OutScaling=2^0
  iDC : Inport  Port=3  OutDataType=sfix(16)  OutScaling=2^0
  I2Q : S-Function  FunctionName=s_I2Q_DC_OS  Parameters="[L  IL0 C  VC0  R]"  EnableBusSupport=off
  Mux1 : Mux  Inputs=3
  "iT1, iD1" : Outport  OutDataType=sfix(16)  OutScaling=2^0
  "iT2, iD2" : Outport  Port=2  OutDataType=sfix(16)  OutScaling=2^0
  iL1 : Outport  Port=3  OutDataType=sfix(16)  OutScaling=2^0
  vC : Outport  Port=4  OutDataType=sfix(16)  OutScaling=2^0
  iE : Outport  Port=5  OutDataType=sfix(16)  OutScaling=2^0
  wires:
  I2Q/5 -> iE/1
  I2Q/3 -> iL1/1
  I2Q/4 -> vC/1
  iDC/1 -> Mux1/3
  I2Q/2 -> "iT2, iD2"/1
  I2Q/1 -> "iT1, iD1"/1
  E/1 -> Mux1/2
  sw/1 -> Mux1/1
  Mux1/1 -> I2Q/1

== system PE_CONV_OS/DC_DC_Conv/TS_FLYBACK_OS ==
  sw : Inport  OutDataType=sfix(16)  OutScaling=2^0
  E : Inport  Port=2  OutDataType=sfix(16)  OutScaling=2^0
  ID : Inport  Port=3  OutDataType=sfix(16)  OutScaling=2^0
  Mux1 : Mux  Inputs=3
  TS_Flyback : S-Function  FunctionName=s_TS_flyback_OS  Parameters="[L1  L2   KP  C  UC0  R]"  EnableBusSupport=off
  iT1 : Outport  OutDataType=sfix(16)  OutScaling=2^0
  iD1 : Outport  Port=2  OutDataType=sfix(16)  OutScaling=2^0
  iT2 : Outport  Port=3  OutDataType=sfix(16)  OutScaling=2^0
  iD2 : Outport  Port=4  OutDataType=sfix(16)  OutScaling=2^0
  iD3 : Outport  Port=5  OutDataType=sfix(16)  OutScaling=2^0
  vC : Outport  Port=6  OutDataType=sfix(16)  OutScaling=2^0
  iE : Outport  Port=7  OutDataType=sfix(16)  OutScaling=2^0
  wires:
  TS_Flyback/7 -> iE/1
  ID/1 -> Mux1/3
  TS_Flyback/6 -> vC/1
  TS_Flyback/5 -> iD3/1
  TS_Flyback/4 -> iD2/1
  TS_Flyback/3 -> iT2/1
  TS_Flyback/2 -> iD1/1
  TS_Flyback/1 -> iT1/1
  E/1 -> Mux1/2
  Mux1/1 -> TS_Flyback/1
  sw/1 -> Mux1/1

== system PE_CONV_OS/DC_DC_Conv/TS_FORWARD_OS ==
  sw : Inport  OutDataType=sfix(16)  OutScaling=2^0
  E : Inport  Port=2  OutDataType=sfix(16)  OutScaling=2^0
  IDC : Inport  Port=3  OutDataType=sfix(16)  OutScaling=2^0
  Mux1 : Mux  Inputs=3
  TS_Forward : S-Function  FunctionName=s_TS_forward_OS  Parameters="[L1  L2   KP  L iL0  C  UC0  R]"  EnableBusSupport=off
  iT1 : Outport  OutDataType=sfix(16)  OutScaling=2^0
  iD1 : Outport  Port=2  OutDataType=sfix(16)  OutScaling=2^0
  iT2 : Outport  Port=3  OutDataType=sfix(16)  OutScaling=2^0
  iD2 : Outport  Port=4  OutDataType=sfix(16)  OutScaling=2^0
  iL1 : Outport  Port=5  OutDataType=sfix(16)  OutScaling=2^0
  vC : Outport  Port=6  OutDataType=sfix(16)  OutScaling=2^0
  iE : Outport  Port=7  OutDataType=sfix(16)  OutScaling=2^0
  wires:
  TS_Forward/7 -> iE/1
  IDC/1 -> Mux1/3
  TS_Forward/6 -> vC/1
  TS_Forward/5 -> iL1/1
  TS_Forward/4 -> iD2/1
  TS_Forward/3 -> iT2/1
  TS_Forward/2 -> iD1/1
  TS_Forward/1 -> iT1/1
  E/1 -> Mux1/2
  Mux1/1 -> TS_Forward/1
  sw/1 -> Mux1/1

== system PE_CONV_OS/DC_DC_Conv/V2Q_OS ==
  sw : Inport  OutDataType=sfix(16)  OutScaling=2^0
  E : Inport  Port=2  OutDataType=sfix(16)  OutScaling=2^0
  EL : Inport  Port=3  OutDataType=sfix(16)  OutScaling=2^0
  Gain : Gain  Gain=-1  ParameterDataType=sfix(16)  ParameterScaling=2^0  OutDataType=sfix(16)  OutScaling=2^0
  I2Q : S-Function  FunctionName=s_V2Q_DC_OS  Parameters="[L  IL0 C  VC0  R]"  EnableBusSupport=off
  Mux1 : Mux  Inputs=3
  "iT1, iD1" : Outport  OutDataType=sfix(16)  OutScaling=2^0
  "iT2, iD2" : Outport  Port=2  OutDataType=sfix(16)  OutScaling=2^0
  vO : Outport  Port=3  OutDataType=sfix(16)  OutScaling=2^0
  iL : Outport  Port=4  OutDataType=sfix(16)  OutScaling=2^0
  vC : Outport  Port=5  OutDataType=sfix(16)  OutScaling=2^0
  iE : Outport  Port=6  OutDataType=sfix(16)  OutScaling=2^0
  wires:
  Gain/1 -> iE/1
  I2Q/3 -> vO/1
  I2Q/4 -> iL/1
  I2Q/6 -> Gain/1
  I2Q/5 -> vC/1
  EL/1 -> Mux1/3
  I2Q/2 -> "iT2, iD2"/1
  I2Q/1 -> "iT1, iD1"/1
  E/1 -> Mux1/2
  sw/1 -> Mux1/1
  Mux1/1 -> I2Q/1

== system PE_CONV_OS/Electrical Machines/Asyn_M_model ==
  Iabc : Inport
  wm : Inport  Port=2
  Psi* : Inport  Port=3
  Fcn : Fcn  Expr=(u[1]*LM*RR/(LLR+LM)) / (u(2)+1e-3)
  G1 : Gain  Gain=1.5*P*LM/(LLR+LM)
  G2 : Gain  Gain=P
  I : Integrator
  I1 : Subsystem
  M : Math  Operator=mod
  Mux : Mux  Inputs=2
  P : Product
  Sum : Sum  Inputs=|++
  T : Terminator
  TF : TransferFcn  Numerator=[LM]  Denominator="[(LLR+LM)/RR   1]"
  abc/dq0k : Subsystem
  c1 : Constant  Value=2*pi
  Te : Outport
  Theta : Outport  Port=2
  Id : Outport  Port=3
  Iq : Outport  Port=4
  Id* : Outport  Port=5
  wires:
  abc/dq0k/3(0k) -> T/1
  I1/1(Id*) -> Id*/1
  Psi*/1 -> I1/1(Phir*)
  Fcn/1 -> Sum/1
  Mux/1 -> Fcn/1
  M/1 -> abc/dq0k/2(th), Theta/1
  c1/1 -> M/2
  I/1 -> M/1
  Sum/1 -> I/1
  G2/1 -> Sum/2
  wm/1 -> G2/1
  G1/1 -> Te/1
  P/1 -> G1/1
  abc/dq0k/2(qk) -> Iq/1, Mux/1, P/2
  TF/1 -> P/1, Mux/2
  abc/dq0k/1(dk) -> Id/1, TF/1
  Iabc/1 -> abc/dq0k/1(abc)

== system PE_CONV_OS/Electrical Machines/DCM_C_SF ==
  va : Inport  OutDataType=sfix(16)  OutScaling=2^0
  TL : Inport  Port=2  OutDataType=sfix(16)  OutScaling=2^0
  vf : Inport  Port=3  OutDataType=sfix(16)  OutScaling=2^0
  Mux2 : Mux  Inputs=3
  tdcm : S-Function  FunctionName=s_DCM_OS  Parameters="[Ra La  Rf Lf If0 Laf J D W0]"  EnableBusSupport=off
  Ia : Outport  OutDataType=sfix(16)  OutScaling=2^0
  emf : Outport  Port=2  OutDataType=sfix(16)  OutScaling=2^0
  TE : Outport  Port=3  OutDataType=sfix(16)  OutScaling=2^0
  W : Outport  Port=4  OutDataType=sfix(16)  OutScaling=2^0
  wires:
  tdcm/3 -> TE/1
  tdcm/2 -> emf/1
  TL/1 -> Mux2/3
  vf/1 -> Mux2/2
  tdcm/4 -> W/1
  va/1 -> Mux2/1
  tdcm/1 -> Ia/1
  Mux2/1 -> tdcm/1

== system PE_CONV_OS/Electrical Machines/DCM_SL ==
  Va : Inport  OutDataType=sfix(16)  OutScaling=2^0
  Tl : Inport  Port=2  OutDataType=sfix(16)  OutScaling=2^0
  Vf : Inport  Port=3  OutDataType=sfix(16)  OutScaling=2^0
  Arm. : TransferFcn  Denominator="[La   Ra]"
  Gain : Gain  Orientation=left  Gain=D  ParameterDataType=sfix(16)  ParameterScaling=2^0  OutDataType=sfix(16)  OutScaling=2^0
  Gain1 : Gain  Gain=Laf  ParameterDataType=sfix(16)  ParameterScaling=2^0  OutDataType=sfix(16)  OutScaling=2^0
  Gain2 : Gain  Gain=1/Lf  ParameterDataType=sfix(16)  ParameterScaling=2^0  OutDataType=sfix(16)  OutScaling=2^0
  Gain3 : Gain  Orientation=left  Gain=Rf  ParameterDataType=sfix(16)  ParameterScaling=2^0  OutDataType=sfix(16)  OutScaling=2^0
  Gain4 : Gain  Gain=1/J  ParameterDataType=sfix(16)  ParameterScaling=2^0  OutDataType=sfix(16)  OutScaling=2^0
  I1 : Integrator  InitialConditionSource=external
  If0 : Constant  Value=If0  OutDataType=sfix(16)  OutScaling=2^0
  Integrator : Integrator  InitialConditionSource=external
  P : Product  OutDataType=sfix(16)  OutScaling=2^0
  P1 : Product  Orientation=left  OutDataType=sfix(16)  OutScaling=2^0
  Sum : Sum  Inputs=|+-  OutDataType=sfix(16)  OutScaling=2^0
  Sum1 : Sum  Inputs=-+-  OutDataType=sfix(16)  OutScaling=2^0
  Sum2 : Sum  Inputs=|+-  OutDataType=sfix(16)  OutScaling=2^0
  omm : Constant  Value=omm0
  ia : Outport
  emf : Outport  Port=2
  Te : Outport  Port=3
  w : Outport  Port=4
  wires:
  omm/1 -> I1/2
  Gain4/1 -> I1/1
  Gain3/1 -> Sum2/2
  If0/1 -> Integrator/2
  Gain2/1 -> Integrator/1
  Integrator/1 -> Gain3/1, Gain1/1
  Sum2/1 -> Gain2/1
  Vf/1 -> Sum2/1
  Gain1/1 -> P/2, P1/1
  Va/1 -> Sum/1
  Gain/1 -> Sum1/3
  Tl/1 -> Sum1/1
  Sum/1 -> Arm./1
  Sum1/1 -> Gain4/1
  Arm./1 -> P/1, ia/1
  P/1 -> Sum1/2, Te/1
  P1/1 -> Sum/2, emf/1
  I1/1 -> w/1, Gain/1, P1/2

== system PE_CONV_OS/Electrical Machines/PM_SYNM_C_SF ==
  Vabc : Inport  OutDataType=sfix(16)  OutScaling=2^0
  TL : Inport  Port=2  OutDataType=sfix(16)  OutScaling=2^0
  PSI : Inport  Port=3  OutDataType=sfix(16)  OutScaling=2^0
  Mux : Mux  Inputs=[3 1 1]
  PM_Sym : S-Function  FunctionName=s_PM_Synm_OS  Parameters=[R1 Lq Ld P J D W0]  EnableBusSupport=off
  Iabc : Outport  OutDataType=sfix(16)  OutScaling=2^0
  TE : Outport  Port=2  OutDataType=sfix(16)  OutScaling=2^0
  Wm : Outport  Port=3  OutDataType=sfix(16)  OutScaling=2^0
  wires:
  PSI/1 -> Mux/3
  TL/1 -> Mux/2
  Vabc/1 -> Mux/1
  Mux/1 -> PM_Sym/1
  PM_Sym/3 -> Wm/1
  PM_Sym/2 -> TE/1
  PM_Sym/1 -> Iabc/1

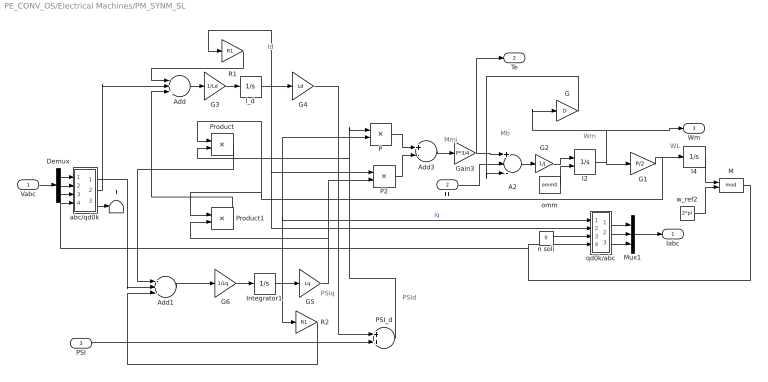
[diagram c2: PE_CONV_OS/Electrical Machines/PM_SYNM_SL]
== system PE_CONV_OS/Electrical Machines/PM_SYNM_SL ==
  note: Mb
  note: Mmi
  note: Wm
  note: WL
  note: PSIq
  note: Id
  note: PSId
  Vabc : Inport
  TL : Inport  Port=2
  PSI : Inport  Port=3
  A2 : Sum  Inputs=+--
  Add : Sum  Inputs=-++
  Add1 : Sum  Inputs=-+-
  Add3 : Sum  Inputs=+-
  Demux : Demux  Outputs=3
  G : Gain  Gain=D
  G1 : Gain  Gain=P/2
  G2 : Gain  Gain=1/J
  G3 : Gain  Gain=1/Ld
  G4 : Gain  Gain=Ld
  G5 : Gain  Gain=Lq
  G6 : Gain  Gain=1/Lq
  Gain3 : Gain  Gain=P*3/4
  I2 : Integrator  InitialConditionSource=external
  I4 : Integrator
  I_d : Integrator
  Integrator1 : Integrator
  M : Math  Operator=mod
  Mux1 : Mux  Inputs=3
  P : Product
  P2 : Product
  PSI_d : Sum
  Product : Product
  Product1 : Product
  R1 : Gain  Gain=R1
  R2 : Gain  Gain=R1
  T : Terminator
  abc/qd0k : Subsystem
  n soll : Constant  Value=0
  omm : Constant  Value=omm0
  qd0k/abc : Subsystem
  w_ref2 : Constant  Value=2*pi
  Iabc : Outport
  Te : Outport  Port=2
  Wm : Outport  Port=3
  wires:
  G/1 -> A2/3
  omm/1 -> I2/2
  abc/qd0k/2(dk) -> Add/2
  M/1 -> qd0k/abc/4(th), abc/qd0k/4(th)
  w_ref2/1 -> M/2
  TL/1 -> A2/2
  I4/1 -> M/1
  Add1/1 -> G6/1
  Integrator1/1 -> R2/1, qd0k/abc/1(qk), P/2, G5/1  "Iq"
  Add/1 -> G3/1
  I_d/1 -> R1/1, qd0k/abc/2(dk), P2/1, G4/1
  abc/qd0k/1(qk) -> Add1/2
  P2/1 -> Add3/2
  P/1 -> Add3/1
  Add3/1 -> Gain3/1
  Gain3/1 -> Te/1, A2/1
  Product1/1 -> Add/3
  Product/1 -> Add1/1
  I2/1 -> G/1, Wm/1, G1/1
  G2/1 -> I2/1
  A2/1 -> G2/1
  R2/1 -> Add1/3
  R1/1 -> Add/1
  abc/qd0k/3(0k) -> T/1
  n soll/1 -> qd0k/abc/3(0k)
  G4/1 -> PSI_d/1
  PSI_d/1 -> P/1, Product/2
  G5/1 -> P2/2, Product1/2
  G1/1 -> Product1/1, Product/1, I4/1
  PSI/1 -> PSI_d/2
  Vabc/1 -> Demux/1
  Demux/2 -> abc/qd0k/2(b)
  Demux/1 -> abc/qd0k/1(a)
  Demux/3 -> abc/qd0k/3(c)
  qd0k/abc/2(b) -> Mux1/2
  qd0k/abc/1(a) -> Mux1/1
  qd0k/abc/3(c) -> Mux1/3
  Mux1/1 -> Iabc/1
  G3/1 -> I_d/1
  G6/1 -> Integrator1/1

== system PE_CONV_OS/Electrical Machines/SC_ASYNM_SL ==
  note: wrm1
  Vabc : Inport
  Tl : Inport  Port=2
  G : Gain  Gain=D
  G1 : Gain  Gain=1/J
  G2 : Gain  Gain=P/2
  G4 : Gain  Gain=P/2
  Gd : Ground
  I1 : Integrator  InitialConditionSource=external
  Mux1 : Mux
  Mux2 : Mux
  P : Product
  P1 : Product
  SS : Subsystem
  SS1 : Subsystem
  Sum : Sum  Inputs=+--
  T : Terminator
  Tem1 : Fcn  Expr=3*(P/4)*(u(3)*u(2)-u(1)*u(4))
  omm : Constant  Value=omm0
  qd0s/abc : Subsystem
  uds : Fcn  Expr=2/3*((-sqrt(3)/2)*u(2)+(sqrt(3)/2)*u(3))
  uqs : Fcn  Expr=2/3*(u(1)-(u(2)/2)-(u(3)/2))
  ia : Outport
  ib : Outport  Port=2
  ic : Outport  Port=3
  Te : Outport  Port=4
  w : Outport  Port=5
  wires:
  qd0s/abc/3(c) -> ic/1
  qd0s/abc/2(b) -> ib/1
  qd0s/abc/1(a) -> ia/1
  omm/1 -> I1/2
  G1/1 -> I1/1
  Mux2/1 -> T/1
  SS1/5(psidm) -> Mux2/4
  SS1/4(idr) -> Mux2/3
  SS/5(psiqm) -> Mux2/2
  SS/4(iqr) -> Mux2/1
  Mux1/1 -> Tem1/1
  Sum/1 -> G1/1
  G2/1 -> P/2
  G4/1 -> P1/2
  uqs/1 -> SS/1(uqs)
  uds/1 -> SS1/1(uds)
  Vabc/1 -> uqs/1, uds/1
  P1/1 -> SS/2(wr*psidr)
  P/1 -> SS1/2(wr*psiqr)
  I1/1 -> G/1, G4/1, G2/1, w/1
  G/1 -> Sum/3
  SS/2(iqs) -> Mux1/2, qd0s/abc/1(q)
  Tem1/1 -> Sum/1, Te/1
  Tl/1 -> Sum/2
  SS/1(psiqs) -> Mux1/1
  SS/3(psiqr) -> P/1
  SS1/3(psidr) -> P1/1
  SS1/2(ids) -> Mux1/4, qd0s/abc/2(d)
  SS1/1(psids) -> Mux1/3
  Gd/1 -> qd0s/abc/3(0)

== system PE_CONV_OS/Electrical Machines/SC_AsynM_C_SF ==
  Vabc : Inport  OutDataType=sfix(16)  OutScaling=2^0
  TL : Inport  Port=2  OutDataType=sfix(16)  OutScaling=2^0
  ASYNM_SC_SF : S-Function  FunctionName=s_Asynm_sc_OS  Parameters=[RS LS RR LR LM P J D W0]  EnableBusSupport=off
  Mux : Mux  Inputs=[3 1]
  iA : Outport  OutDataType=sfix(16)  OutScaling=2^0
  iB : Outport  Port=2  OutDataType=sfix(16)  OutScaling=2^0
  iC : Outport  Port=3  OutDataType=sfix(16)  OutScaling=2^0
  TE : Outport  Port=4  OutDataType=sfix(16)  OutScaling=2^0
  W : Outport  Port=5  OutDataType=sfix(16)  OutScaling=2^0
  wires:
  ASYNM_SC_SF/5 -> W/1
  ASYNM_SC_SF/4 -> TE/1
  ASYNM_SC_SF/1 -> iA/1
  ASYNM_SC_SF/3 -> iC/1
  ASYNM_SC_SF/2 -> iB/1
  TL/1 -> Mux/2
  Vabc/1 -> Mux/1
  Mux/1 -> ASYNM_SC_SF/1

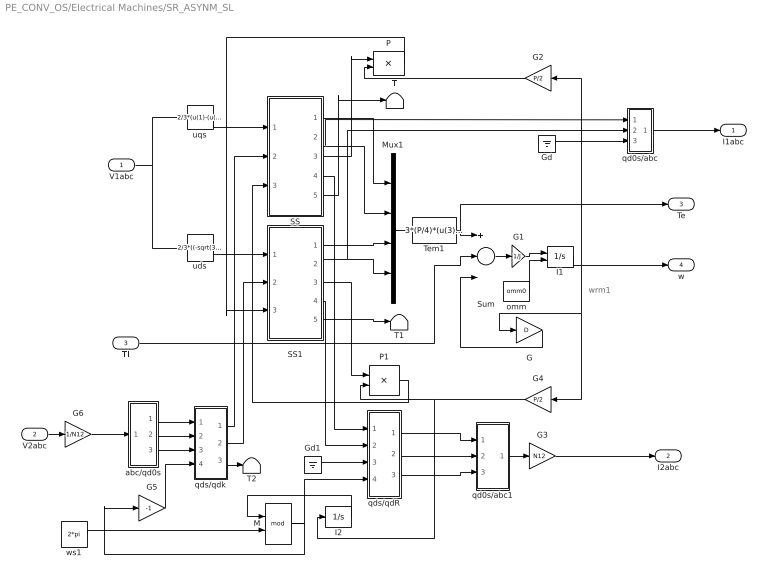
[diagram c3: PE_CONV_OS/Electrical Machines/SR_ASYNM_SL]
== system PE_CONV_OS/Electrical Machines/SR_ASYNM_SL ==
  note: wrm1
  V1abc : Inport
  V2abc : Inport  Port=2
  Tl : Inport  Port=3
  G : Gain  Gain=D
  G1 : Gain  Gain=1/J
  G2 : Gain  Orientation=left  Gain=P/2
  G3 : Gain  Gain=N12
  G4 : Gain  Orientation=left  Gain=P/2
  G5 : Gain  Gain=-1
  G6 : Gain  Gain=1/N12
  Gd : Ground
  Gd1 : Ground
  I1 : Integrator  InitialConditionSource=external
  I2 : Integrator
  M : Math  Operator=mod
  Mux1 : Mux
  P : Product
  P1 : Product
  SS : Subsystem
  SS1 : Subsystem
  Sum : Sum  Inputs=+--
  T : Terminator
  T1 : Terminator
  T2 : Terminator
  Tem1 : Fcn  Expr=3*(P/4)*(u(3)*u(2)-u(1)*u(4))
  abc/qd0s : Subsystem
  omm : Constant  Value=omm0
  qd0s/abc : Subsystem
  qd0s/abc1 : Subsystem
  qds/qdR : Subsystem
  qds/qdk : Subsystem
  uds : Fcn  Expr=2/3*((-sqrt(3)/2)*u(2)+(sqrt(3)/2)*u(3))
  uqs : Fcn  Expr=2/3*(u(1)-(u(2)/2)-(u(3)/2))
  ws1 : Constant  Value=2*pi
  I1abc : Outport
  I2abc : Outport  Port=2
  Te : Outport  Port=3
  w : Outport  Port=4
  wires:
  G6/1 -> abc/qd0s/1(a)
  G3/1 -> I2abc/1
  V2abc/1 -> G6/1
  V1abc/1 -> uds/1, uqs/1
  qds/qdk/2(dk) -> SS1/2(udr)
  qds/qdk/1(qk) -> SS/2(uqr)
  G5/1 -> qds/qdk/4(th)
  abc/qd0s/3(0) -> qds/qdk/3(0s)
  abc/qd0s/1(q) -> qds/qdk/1(qs)
  abc/qd0s/2(d) -> qds/qdk/2(ds)
  M/1 -> qds/qdR/4(th), G5/1
  ws1/1 -> M/2
  I2/1 -> M/1
  Gd1/1 -> qds/qdR/3(0s)
  SS1/4(idr) -> qds/qdR/2(ds)
  SS/4(iqr) -> qds/qdR/1(qs)
  Gd/1 -> qd0s/abc/3(0)
  SS1/1(psids) -> Mux1/3
  SS1/2(ids) -> qd0s/abc/2(d), Mux1/4
  SS1/3(psidr) -> P1/1
  SS/3(psiqr) -> P/1
  SS/1(psiqs) -> Mux1/1
  Tl/1 -> Sum/2
  Tem1/1 -> Te/1, Sum/1
  SS/2(iqs) -> qd0s/abc/1(q), Mux1/2
  G/1 -> Sum/3
  I1/1 -> w/1, G2/1, G4/1, G/1
  P/1 -> SS1/3(wr*ps)
  P1/1 -> SS/3(wr*ps)
  uds/1 -> SS1/1(uds)
  uqs/1 -> SS/1(uqs)
  G4/1 -> I2/1, P1/2
  G2/1 -> P/2
  Sum/1 -> G1/1
  Mux1/1 -> Tem1/1
  qds/qdR/3(0k) -> qd0s/abc1/3(0)
  qds/qdR/2(dk) -> qd0s/abc1/2(d)
  qds/qdR/1(qk) -> qd0s/abc1/1(q)
  qd0s/abc1/1(a) -> G3/1
  qd0s/abc/1(a) -> I1abc/1
  SS/5(psiqm) -> T/1
  SS1/5(psidm) -> T1/1
  qds/qdk/3(0k) -> T2/1
  G1/1 -> I1/1
  omm/1 -> I1/2

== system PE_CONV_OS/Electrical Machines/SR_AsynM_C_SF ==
  V1abc : Inport  OutDataType=sfix(16)  OutScaling=2^0
  V2abc : Inport  Port=2  OutDataType=sfix(16)  OutScaling=2^0
  TL : Inport  Port=3  OutDataType=sfix(16)  OutScaling=2^0
  ASYNM_SC_SF : S-Function  FunctionName=s_Asynm_sr_OS  Parameters="[RS LS RR LR LM  N12  P J D W0]"  EnableBusSupport=off
  Mux : Mux  Inputs="[3  3  1]"
  i1abc : Outport  OutDataType=sfix(16)  OutScaling=2^0
  i2abc : Outport  Port=2  OutDataType=sfix(16)  OutScaling=2^0
  TE : Outport  Port=3  OutDataType=sfix(16)  OutScaling=2^0
  W : Outport  Port=4  OutDataType=sfix(16)  OutScaling=2^0
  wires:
  V2abc/1 -> Mux/2
  TL/1 -> Mux/3
  Mux/1 -> ASYNM_SC_SF/1
  V1abc/1 -> Mux/1
  ASYNM_SC_SF/2 -> i2abc/1
  ASYNM_SC_SF/3 -> TE/1
  ASYNM_SC_SF/1 -> i1abc/1
  ASYNM_SC_SF/4 -> W/1

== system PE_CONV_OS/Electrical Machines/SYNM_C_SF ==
  Vabc : Inport  OutDataType=sfix(16)  OutScaling=2^0
  Vdf : Inport  Port=2  OutDataType=sfix(16)  OutScaling=2^0
  TL : Inport  Port=3  OutDataType=sfix(16)  OutScaling=2^0
  Mux : Mux  Inputs="[3 1   1]"
  SYNM_SC_SF : S-Function  FunctionName=s_Synm_OS  Parameters="[rs Lls rk Llkq  Llkd Lmq Lmd rf  Llf  P J D]"  EnableBusSupport=off
  iA : Outport  OutDataType=sfix(16)  OutScaling=2^0
  iB : Outport  Port=2  OutDataType=sfix(16)  OutScaling=2^0
  iC : Outport  Port=3  OutDataType=sfix(16)  OutScaling=2^0
  TE : Outport  Port=4  OutDataType=sfix(16)  OutScaling=2^0
  W : Outport  Port=5  OutDataType=sfix(16)  OutScaling=2^0
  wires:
  Vdf/1 -> Mux/2
  SYNM_SC_SF/5 -> W/1
  SYNM_SC_SF/4 -> TE/1
  SYNM_SC_SF/1 -> iA/1
  SYNM_SC_SF/3 -> iC/1
  SYNM_SC_SF/2 -> iB/1
  TL/1 -> Mux/3
  Vabc/1 -> Mux/1
  Mux/1 -> SYNM_SC_SF/1

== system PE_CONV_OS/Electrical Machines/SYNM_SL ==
  Vabc : Inport
  Vfd : Inport  Port=2
  Tl : Inport  Port=3
  G : Gain  Gain=D
  G1 : Gain  Gain=1/J
  G2 : Gain  Gain=P/2
  G4 : Gain  Gain=P/2
  Gd : Ground
  Gn : Terminator
  I : Integrator
  I1 : Integrator  InitialConditionSource=external
  Mux1 : Mux
  P : Product
  P1 : Product
  SS : Subsystem
  SS1 : Subsystem
  Sum : Sum  Inputs=+--
  Tem1 : Fcn  Expr=3*(P/4)*(u(3)*u(2)-u(1)*u(4))
  abc/qd0 : Subsystem
  omm : Constant  Value=omm0
  qd0k/abc : Subsystem
  qds/qdk : Subsystem
  ia : Outport
  ib : Outport  Port=2
  ic : Outport  Port=3
  Te : Outport  Port=4
  w : Outport  Port=5
  idf : Outport  Port=6
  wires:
  omm/1 -> I1/2
  G1/1 -> I1/1
  qd0k/abc/3(c) -> ic/1
  I/1 -> qd0k/abc/4(th), qds/qdk/3(th)
  SS1/1(psids) -> Mux1/3, P1/1
  SS1/2(ids) -> qd0k/abc/2(dk), Mux1/4
  Tl/1 -> Sum/2
  Tem1/1 -> Te/1, Sum/1
  SS/2(iqs) -> qd0k/abc/1(qk), Mux1/2
  G/1 -> Sum/3
  I1/1 -> G/1, G4/1, w/1, G2/1
  P1/1 -> SS/2(wr*psids)
  G4/1 -> P1/2
  Sum/1 -> G1/1
  Mux1/1 -> Tem1/1
  abc/qd0/1(q) -> qds/qdk/1(qs)
  abc/qd0/3(0) -> Gn/1
  SS/1(psiqs) -> P/1, Mux1/1
  SS1/7(idf) -> idf/1
  qds/qdk/1(qk) -> SS/1(uqs)
  qds/qdk/2(dk) -> SS1/1(uds)
  Vfd/1 -> SS1/3(udf)
  abc/qd0/2(d) -> qds/qdk/2(ds)
  Vabc/1 -> abc/qd0/1(abc)
  G2/1 -> I/1, P/2
  P/1 -> SS1/2(wr*psiqs)
  qd0k/abc/1(a) -> ia/1
  qd0k/abc/2(b) -> ib/1
  Gd/1 -> qd0k/abc/3(0k)

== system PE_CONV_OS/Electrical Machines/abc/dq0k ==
  a : Inport  OutDataType=sfix(16)  OutScaling=2^0
  b : Inport  Port=2  OutDataType=sfix(16)  OutScaling=2^0
  c : Inport  Port=3  OutDataType=sfix(16)  OutScaling=2^0
  th : Inport  Port=4  OutDataType=sfix(16)  OutScaling=2^0
  Demux : Demux  Outputs=3
  Fcn : Fcn  Expr=u(1)*cos(u(3)) + u(2)*sin(u(3))
  Fcn1 : Fcn  Expr=-u(1)*sin(u(3)) + u(2)*cos(u(3))
  K : Gain  Gain="2/3*[1   -.5   -.5;  0   sqrt(3)/2   -sqrt(3)/2;  .5    .5    .5]"  Multiplication=Matrix(K*u)  ParameterDataType=sfix(16)  ParameterScaling=2^0  OutDataType=sfix(16)  OutScaling=2^0
  Mux : Mux  Inputs=3
  Mux1 : Mux  Inputs=3
  dk : Outport
  qk : Outport  Port=2
  0k : Outport  Port=3
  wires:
  Demux/2 -> Mux1/2
  Demux/1 -> Mux1/1
  Demux/3 -> 0k/1
  th/1 -> Mux1/3
  Fcn1/1 -> qk/1
  Fcn/1 -> dk/1
  Mux1/1 -> Fcn/1, Fcn1/1
  a/1 -> Mux/1
  Mux/1 -> K/1
  K/1 -> Demux/1
  b/1 -> Mux/2
  c/1 -> Mux/3
